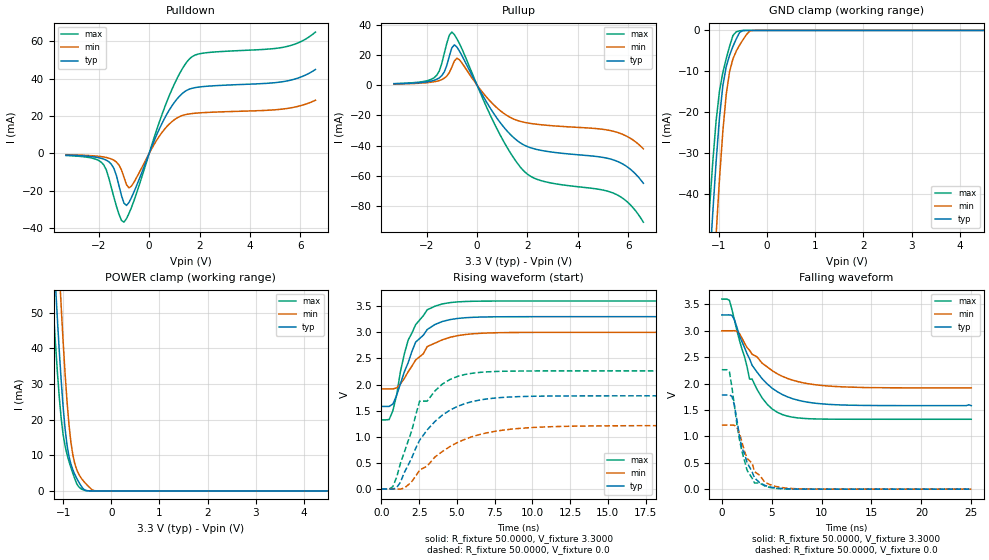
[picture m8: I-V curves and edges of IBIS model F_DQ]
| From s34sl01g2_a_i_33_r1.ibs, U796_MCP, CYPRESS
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|   Model   F_DQ
[Model]   F_DQ
Model_type I/O
Polarity   Non-Inverting
Enable   Active-Low
Vinl =   0.6600V
Vinh =   2.6400V
Vmeas =  1.6500V
Cref =   30.0000pF
   C_comp   0.5220pF   0.5218pF   0.5220pF
[Temperature Range]   25.0000   0.1050k   -40.0000
[Pullup Reference]   3.3000V   3.0000V   3.6000V
[Pulldown Reference]   0.0V   0.0V   0.0V
[POWER Clamp Reference]   3.3000V   3.0000V   3.6000V
[GND Clamp Reference]   0.0V   0.0V   0.0V
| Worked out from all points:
|   slope of the pulldown table from 0 to 0.495 V, typ, clamps not added: 31.5 ohm
|   slope of the pullup table from 0 to 0.495 V, typ, clamps not added: 34.2 ohm
|   GND clamp passes 1 mA (typ) near -0.59 V on its own axis
|   POWER clamp passes 1 mA (typ) near -0.61 V on its own axis
|   rising waveform, R_fixture 50.0000, V_fixture 3.3000: 20-80 % time 1.65ns typ, 1.92ns min, 1.28ns max; typ from 1.58 V to 3.3 V
|   rising waveform, R_fixture 50.0000, V_fixture 0.0: 20-80 % time 2.51ns typ, 3.45ns min, 2.14ns max; typ from 0 V to 1.78 V
|   falling waveform, R_fixture 50.0000, V_fixture 3.3000: 20-80 % time 3.28ns typ, 3.87ns min, 2.54ns max; typ from 3.3 V to 1.58 V
|   falling waveform, R_fixture 50.0000, V_fixture 0.0: 20-80 % time 1.55ns typ, 1.97ns min, 1.3ns max; typ from 1.78 V to 0 V
[Pulldown]
|Voltage   I(typ)   I(min)   I(max)
-3.3V     -870uA     -670uA     -1.1mA
-1.8V     -3.03mA    -1.91mA    -6.19mA
-1.4V     -7.99mA    -3.62mA    -23.39mA
-1.2V     -17.13mA   -6.147mA   -32.49mA
-1V       -26.58mA   -12.7mA    -36.8mA
-800mV    -26.23mA   -18.42mA   -32.1mA
-700mV    -23.56mA   -17.44mA   -28.86mA
600mV     18.51mA    12.81mA    24.16mA
1.1V      29.07mA    18.96mA    39.96mA
1.6V      34.46mA    21.2mA     50.63mA
5.4V      38.66mA    23.95mA    57.08mA
6.6V      44.96mA    28.5mA     64.99mA
[Pullup]
|Voltage   I(typ)   I(min)   I(max)
-3.3V     880uA      710uA      1mA
-1.7V     3.24mA     2.25mA     4.97mA
-1.5V     4.8mA      3.03mA     9.37mA
-1.3V     8.784mA    4.6mA      21.11mA
-1V       24.75mA    11.96mA    35.12mA
-700mV    22.53mA    16.78mA    27.52mA
700mV     -19.73mA   -13.66mA   -25.95mA
1.9V      -39.97mA   -24.7mA    -57.56mA
2.7V      -43.67mA   -26.48mA   -63.95mA
5.4V      -49.45mA   -30.5mA    -71.44mA
6V        -54.58mA   -34.37mA   -77.87mA
6.6V      -64.99mA   -42.19mA   -90.75mA
[GND_clamp]
|Voltage   I(typ)   I(min)   I(max)
-3.3V     -533.4mA   -612.6mA   -471.4mA
-1.27V    -72.49mA   -96.24mA   -56.66mA
-1.2V     -58.24mA   -80.16mA   -43.99mA
-1.13V    -44.63mA   -64.63mA   -32.2mA
-1.06V    -32.08mA   -49.87mA   -22.07mA
-990mV    -21.33mA   -36.29mA   -14.79mA
-920mV    -13.5mA    -24.59mA   -10.27mA
-850mV    -8.877mA   -15.65mA   -6.884mA
-780mV    -6.057mA   -10.04mA   -3.875mA
-640mV    -2.044mA   -5.019mA   -322.1uA
-290mV    -134.5nA   -20.19uA   -70.42nA
6.6V      202.3pA    18.45uA    151.9pA
[POWER_clamp]
|Voltage   I(typ)   I(min)   I(max)
-3.28V    693.8mA    805.9mA    602.9mA
-1.24V    78.63mA    108mA      59.13mA
-1.2V     68.14mA    96.01mA    50.03mA
-1.16V    57.99mA    84.27mA    41.37mA
-1.12V    48.27mA    72.87mA    33.33mA
-1.08V    39.13mA    61.91mA    26.18mA
-1.04V    30.77mA    51.49mA    20.25mA
-920mV    12.92mA    25.17mA    10.25mA
-800mV    5.975mA    10.18mA    4.993mA
-600mV    882.5uA    3.143mA    384.7uA
-280mV    290.9nA    10.18uA    181.8nA
6.6V      202.3pA    4.26nA     189.5pA
[Ramp]
| variable   typ   min   max
dV/dt_r  1.0706/2.5732n   0.7283/3.2643n   1.3573/1.9850n
dV/dt_f  1.0310/3.2797n   0.6493/3.5324n   1.3657/2.5101n
R_load = 50.0000
[Rising Waveform]
R_fixture= 50.0000
V_fixture= 3.3000
V_fixture_min= 3.0000
V_fixture_max= 3.6000
|time   V(typ)   V(min)   V(max)
0s        1.582V     1.918V     1.324V
510ps     1.581V     1.918V     1.33V
760ps     1.628V     1.917V     1.503V
1.26ns    2.016V     2.01V      2.251V
1.77ns    2.419V     2.245V     2.85V
2.27ns    2.814V     2.472V     3.149V
3.03ns    3.054V     2.727V     3.431V
3.54ns    3.149V     2.793V     3.5V
7.07ns    3.296V     2.988V     3.598V
25ns      3.3V       3V         3.6V
[Rising Waveform]
R_fixture= 50.0000
V_fixture= 0.0
V_fixture_min= 0.0
V_fixture_max= 0.0
|time   V(typ)   V(min)   V(max)
0s        -228.3nV   168.1nV    -593.2nV
760ps     -2.357mV   -88.28uV   46.48mV
1.26ns    130mV      -1.669mV   495.4mV
1.52ns    319.2mV    20.89mV    707.8mV
2.53ns    935.4mV    363.2mV    1.683V
3.03ns    1.132V     439.9mV    1.683V
3.54ns    1.292V     612.4mV    1.878V
5.05ns    1.584V     893.2mV    2.157V
10.1ns    1.776V     1.179V     2.261V
25ns      1.784V     1.214V     2.262V
[Falling Waveform]
R_fixture= 50.0000
V_fixture= 3.3000
V_fixture_min= 3.0000
V_fixture_max= 3.6000
|time   V(typ)   V(min)   V(max)
0s        3.3V       3V         3.6V
760ps     3.3V       3V         3.576V
1.01ns    3.292V     3V         3.405V
1.52ns    3.061V     2.991V     2.995V
2.78ns    2.469V     2.629V     2.085V
3.03ns    2.348V     2.556V     2.085V
4.04ns    2.092V     2.385V     1.728V
5.56ns    1.845V     2.185V     1.456V
10.1ns    1.614V     1.962V     1.327V
25ns      1.582V     1.918V     1.324V
[Falling Waveform]
R_fixture= 50.0000
V_fixture= 0.0
V_fixture_min= 0.0
V_fixture_max= 0.0
|time   V(typ)   V(min)   V(max)
0s        1.784V     1.214V     2.262V
760ps     1.784V     1.214V     2.224V
1.26ns    1.594V     1.21V      1.577V
2.02ns    774mV      890.3mV    712.7mV
2.53ns    505.7mV    582.4mV    357.9mV
3.03ns    330.1mV    493.5mV    209.5mV
3.28ns    212.1mV    331.9mV    116.2mV
4.8ns     42.46mV    87.57mV    32.85mV
6.82ns    4.817mV    14.8mV     2.584mV
25ns      -45.34nV   133.6nV    -140.9nV
